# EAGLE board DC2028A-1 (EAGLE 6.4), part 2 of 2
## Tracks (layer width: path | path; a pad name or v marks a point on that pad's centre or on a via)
+3V3  (via drill 0.25)
  Top 0.203: R35.1 61.63,5.5 61.47,5.71 59.56,5.71 59.56,7.49 59.33,7.47 R24.R1_2 | U8.8 59.52,12.99 59.56,12.95 v58.67,12.95 | 66.42,11.81 U13.18 | R25.1 71.63,7.87 71.63,7.37 71.37,7.11 69.98,7.11 69.72,7.37 69.72,10.67 69.09,11.3 69.09,12.19 | C18.2 45.81,19.52 v45.85,19.56 | v45.85,19.56 45.85,20.2 U6.16 | U6.17 45.9,19.5 v45.85,19.56 | v45.85,19.56 45.85,19.5
  Top 0.305: U8.8 59.82,12.95 59.82,11.94 59.8,11.92 59.5,11.92 C20.1 R24.R4_2
  Top 0.406: R24.R1_2 R24.R2_2 R24.R3_2 R24.R4_2 | 66.42,11.81 66.8,12.19 69.09,12.19 69.09,12.83 v69.34,13.08 | R23.2 R22.2 R18.2 57.37,19.47 v57.15,19.68
  Route15 0.406: v69.34,13.08 69.34,12.7 68.96,12.32 67.82,12.32 67.44,11.94 60.81,11.94 U8.8 58.72,12.99 v58.67,12.95 | v24.38,19.94 24.38,17.78 24.51,17.65 45.47,17.65 45.85,18.03 v45.85,19.56
  Bottom 0.203: R60.1 R58.1 68.71,16.6 68.71,14.86 | 68.71,14.86 69.34,14.22 v69.34,13.08 | R67.1 23.07,25.78 | R57.1 67.4,14.31 67.44,14.35 67.44,14.86 68.71,14.86
  Bottom 0.406: v58.67,12.95 58.67,13.59 57.02,15.24 56.32,15.24 R59.R1_2 R59.R2_2 R59.R3_2 R59.R4_2 56.64,17.91 57.15,18.41 v57.15,19.68 57.15,20.32 57.02,20.45 55.88,20.45 55.37,19.94 45.85,19.94 v45.85,19.56 | U16.5 19.81,23.62 19.56,23.88 19.56,25.78 C46.1 23.07,25.78 | R62.2 23.33,20.49 | R62.2 23.37,20.57 | 24.38,20.45 24.51,20.45 24.51,25.27 24.26,25.53 23.41,25.53 R67.1 | v24.38,19.94 24.38,20.45 | R62.2 23.2,20.45 23.2,20.41 23.24,20.45 24.38,20.45
+12V
  Route15 1.016: JP2.14 JP2.13
  pour Top (no thermals): 63.63,30.3 63.63,32.77 72.64,32.77 73.66,33.78 76.07,33.78 77.34,32.64 77.34,30.23 75.82,28.7 68.58,28.7 68.58,29.59 67.82,30.35 65.53,30.35
  pour Bottom (no thermals): 70.61,26.42 70.61,36.45 71.25,37.08 71.25,41.78 71.63,42.16 73.41,42.16 73.79,41.78 73.79,34.29 74.17,33.91 76.07,33.91 77.22,32.89 77.22,30.1 75.56,28.45 75.56,21.08 73.03,18.54 73.03,3.81 72.52,3.3 70.36,3.3 70.36,23.88 72.64,23.88 72.64,26.42
A0_MUX  (via drill 0.25)
  Top 0.203: U13.3 63.37,8.76 62.94,8.38 62.79,8.38 v62.79,8.46 62.79,8.41 62.76,8.38 62.34,8.38 | 62.34,8.38 R24.R2_1 62.08,8.36 62.1,8.38 62.34,8.38
  Bottom 0.203: v62.79,8.46 62.79,8.41 62.76,8.38 61.98,8.38 61.47,7.87 JP3.6
A1_MUX  (via drill 0.25)
  Top 0.203: U13.2 64.16,9.27 63.42,9.27 63.28,9.16 R24.R3_1 61.61,9.16 61.59,9.14 62.79,9.14 | 62.79,9.14 62.9,9.16 | 62.79,9.14 v62.79,9.45 62.79,9.27
  Bottom 0.203: v62.79,9.45 61.9,9.45 61.59,9.14 JP3.7
A2_MUX  (via drill 0.25)
  Top 0.203: 62.79,10.16 63.88,10.16 63.88,9.78 64.14,9.78 U13.1 | R24.R4_1 61.94,10.12 61.98,10.16 62.79,10.16 | 62.79,10.16 v62.79,10.54
  Bottom 0.203: v62.79,10.54 60.71,10.54 JP3.8
ALERTB  (via drill 0.25)
  Top 0.203: v58.42,16.51 58.42,15.11 58.04,14.73 55.63,14.73 | 55.63,14.73 54.48,14.73 53.85,15.37 53.85,16.13 52.7,17.27 v52.32,17.27 52.54,17.31 U6.29 | 55.63,15.62 55.65,15.6 | 55.63,14.73 55.63,15.62 | 55.63,15.62 R23.1
  Route15 0.203: v21.21,18.92 21.21,16.76 48.64,16.76 48.9,17.02 51.05,17.02 51.31,17.27 v52.32,17.27
  Bottom 0.203: JP1.3 62.04,38.42 61.72,38.1 60.58,38.1 59.05,36.58 59.05,33.53 58.93,33.4 58.93,20.95 59.82,20.07 59.82,16.51 | 59.82,16.51 59.82,14.61 60.2,14.22 60.2,12.19 60.45,11.94 62.48,11.94 63.63,10.79 63.63,8.26 61.98,6.6 61.98,3.78 JP2.3 | v58.42,16.51 59.82,16.51 | TP10.TP 15.49,26.92 16.38,26.04 16.38,23.37 16.76,22.99 18.31,22.99 U16.1 18.54,22.99 18.58,22.95 18.58,20.41 20.07,18.92 v21.21,18.92 20.95,18.92
CH7_SHORT  (via drill 0.25)
  Top 0.406: v13.59,24 13.59,18.72 SW2.SW1
  Route15 0.203: v13.59,24 13.59,23.62 8,23.62 6.6,22.23 6.6,16.89 9.27,14.22 12.06,14.22 13.46,15.62 48.51,15.62 49.28,14.86 v51.31,14.86
  Bottom 0.203: Q5.1 53.07,13.1 52.45,13.72 51.56,13.72 51.31,13.97 v51.31,14.86
  Bottom 0.406: R68.2 13.59,25.27 v13.59,24 13.59,19.94 R61.2
CTRL  (via drill 0.25)
  Top 0.203: C26.1 70.74,10.03 71.12,10.41 72.52,10.41 72.77,10.67 S1.5 | U6.31 U6.30 | U6.31 53.34,19.43 | 54.74,18.54 54.74,19.56 54.86,19.68 55.37,19.68 56.01,20.32 56.26,20.32 56.77,20.83 v57.91,20.83 | U6.31 53.41,19.5 53.34,19.43 53.34,18.54 54.74,18.54 | R22.1 54.74,17.14 54.74,18.54
  Top 0.406: S1.2 S1.5
  Route15 0.203: S1.5 | v58.8,18.8 59.18,18.41 59.18,17.27 60.71,15.75 65.15,15.75 65.79,16.38 72.39,16.38 72.77,16 S1.2
  Bottom 0.203: R88.2 59.48,42.08 58.93,41.53 58.93,41.15 | 58.93,41.15 60.02,41.15 JP1.2 58.94,41.13 58.93,41.15 | 58.93,41.15 58.93,37.72 58.29,37.08 58.29,34.04 58.17,33.78 58.17,20.95 58.04,20.83 | 58.04,18.8 58.04,18.54 57.4,17.91 57.4,15.75 59.44,13.72 59.44,12.45 59.18,12.19 59.18,5.21 58.8,4.83 58.8,2.03 59.05,1.78 59.98,1.78 JP2.2 | 58.04,18.8 58.04,20.83 | 58.04,20.83 v57.91,20.83 | 58.04,18.8 v58.8,18.8
CTRL_P
  Bottom 0.203: R88.1 61.17,43.22 61.21,43.18 66.04,43.18 67.03,42.19 67.03,38.38 68.33,37.08 TP8.TP
DACP_CH0  (via drill 0.25)
  Top 0.203: U6.39 55.49,23.25 v55.75,22.99
  Route15 0.203: v55.75,22.99 55.24,22.99 54.99,23.24 54.99,23.5 54.99,23.88 53.59,25.27 48.39,25.27 47.5,26.16 42.67,26.16 41.4,27.43 33.53,27.43 32.77,28.19 32.77,30.61 31.88,31.5 21.97,31.5 21.72,31.75 VSNSN23.1
  Bottom 0.203: R78.2 21.97,33.91 21.72,33.91
  Bottom 0.406: VSNSN23.1 21.72,33.91
DACP_CH1  (via drill 0.25)
  Top 0.203: U6.40 55.63,23.75 v55.75,23.88
  Route15 0.203: v55.75,23.88 53.98,25.65 48.64,25.65 47.75,26.54 42.93,26.54 41.66,27.81 33.78,27.81 33.27,28.32 VSNSN21.1
  Bottom 0.203: R76.2 33.53,33.91 33.27,33.91
  Bottom 0.406: VSNSN21.1 33.27,33.91
DACP_CH2  (via drill 0.25)
  Top 0.203: U6.44 55.27,25.75 55.37,25.65 56.64,25.65 56.77,25.53 v56.77,25.02
  Route15 0.203: v56.77,25.02 56.77,25.53 56.64,25.65 55.5,25.65 54.61,26.54 49.02,26.54 47.37,28.19 47.37,29.72 VSNSN19.1
  Bottom 0.203: R74.2 45.09,33.91 44.83,33.91
  Bottom 0.406: VSNSN19.1 44.83,33.91
DACP_CH3  (via drill 0.25)
  Top 0.203: U6.50 53.54,29.16 53.72,29.34 55.24,29.34 55.37,29.34 55.63,29.08 55.63,28.7 v55.75,28.7
  Bottom 0.203: R72.2 56.64,33.91 56.39,33.91 | v55.75,28.7 55.63,28.7 55.63,31.88 55.88,32.26 VSNSN17.1
  Bottom 0.406: VSNSN17.1 56.39,33.91
DACP_CH4  (via drill 0.25)
  Top 0.203: U6.55 51.04,29.07 51.31,29.34 52.2,29.34 53.09,30.23 56.13,30.23 57.02,29.34 57.02,28.07 56.64,27.69 v56.64,27.56
  Route15 0.203: v56.64,27.56 56.64,27.43 57.4,26.67 57.4,22.61 55.88,21.08 47.62,21.08 45.72,22.99 43.94,22.99 43.18,22.23 43.18,19.3 43.05,19.18 40.77,19.18 39.5,20.45 26.8,20.45 26.67,20.57 21.08,20.57 20.45,19.94 20.45,17.27 14.22,17.27 v14.22,17.4
  Bottom 0.203: R56.2 13.21,12.45 13.46,12.45 | VSNSN16.1 13.72,17.14 13.97,17.4 v14.22,17.4
  Bottom 0.406: 13.46,12.45 13.72,12.45 VSNSN16.1
DACP_CH5  (via drill 0.25)
  Top 0.203: U6.56 50.54,29.21 51.05,29.72 51.94,29.72 52.83,30.61 56.39,30.61 57.53,29.46 v57.53,27.56
  Route15 0.203: v57.53,27.56 57.53,27.18 57.78,26.92 57.78,22.35 56.13,20.7 47.37,20.7 45.47,22.61 44.2,22.61 43.69,22.1 43.69,19.05 43.31,18.67 40.64,18.67 39.37,19.94 v26.16,19.94
  Bottom 0.203: R54.2 24.77,12.45 25.02,12.45 | v26.16,19.94 26.16,15.24 VSNSN14.1
  Bottom 0.406: 25.02,12.45 VSNSN14.1
DACP_CH6  (via drill 0.25)
  Top 0.203: U6.59 49.04,29.32 48.64,29.72 48.26,29.72 47.75,30.23 45.09,30.23 44.45,29.59 v44.45,29.34 | VSNSN12.1 36.58,18.16 36.58,18.41 36.83,18.67 v37.72,18.67
  Bottom 0.203: R52.2 36.32,12.45 36.58,12.45 | v44.45,29.34 43.43,29.34 42.16,28.07 42.16,25.78 41.91,25.53 39.5,25.53 38.35,24.38 38.35,19.18 37.85,18.67 v37.72,18.67
  Bottom 0.406: 36.58,12.45 VSNSN12.1
DACP_CH7  (via drill 0.25)
  Top 0.203: U6.60 48.54,29.18 48.39,29.34 48.01,29.34 47.5,29.84 45.47,29.84 v45.47,29.59
  Bottom 0.203: R50.2 47.88,12.45 48.13,12.45 | VSNSN10.1 48.13,14.73 47.88,14.99 44.07,14.99 43.81,15.24 43.81,27.56 44.07,27.81 44.7,27.81 45.47,28.57 v45.47,29.59
  Bottom 0.406: 48.13,12.45 VSNSN10.1
EESCL
  Top 0.203: 77.47,6.1 77.22,6.35 R30.1 78.03,6.35 | U14.1 77.81,1.59 78.03,1.78 78.03,6.35 | 78.03,6.35 78.03,6.66 78.61,7.24 78.61,8 78.87,8.26 83.66,8.26 84.17,8.76 84.17,10.29 83.72,10.73 82.01,10.73 J2.11 81.09,9.65
EESDA
  Top 0.203: 77.21,3.43 U14.3 77.21,4.83 R36.1 76.33,4.83 76.33,7.06 76.45,7.19 77.95,7.19 78.11,7.34 78.11,8.26 78.49,8.64 82.9,8.64 83.19,8.89 83.19,9.65 J2.12
EEVCC  (via drill 0.25)
  Top 0.203: 78.81,20.77 78.2,20.77 C15.1
  Top 0.254: U7.8 U7.7
  Top 0.406: R36.2 R30.2 75.44,6.35 | U14.4 74.36,3.49 74.68,3.56 | 74.68,4.79 R36.2 | 74.68,3.56 74.55,3.56 | 74.68,4.79 74.68,4.83 | 74.68,3.56 74.68,4.79 | R36.2 74.68,4.83 | 74.68,4.83 v74.3,4.83 | 75.44,6.35 75.35,6.35 | 75.44,6.35 75.44,7.87 C25.1
  Top 0.813: 83.95,37.85 84.07,37.59 84.07,22.61 83.95,22.48
  Top 1.016: 83.95,37.85 82.9,38.86 79.63,38.86 78.87,39.62 74.8,39.62 73.53,40.89 73.53,42.55 73.15,42.93 66.55,42.93 66.02,42.4 66.02,41.15 JP1.8 | 79.63,22.48 83.95,22.48 | 79.63,22.48 v79.63,21.84 79.63,21.59 78.81,20.77 U7.8 | 79.63,22.48 v79.63,22.99
  Route15 0.406: v68.07,19.56 69.6,19.56 71.88,21.84 v79.63,21.84
  Bottom 0.406: D1.2 68.98,19.8 68.58,19.56 v68.07,19.56
  Bottom 0.813: J2.1 81.01,19.7 80.99,19.68 79.6,19.68 arc60 79.63,19.81 v79.63,21.84 v79.63,22.99
  pour Bottom (no thermals): 65.28,2.92 72.77,2.92 73.53,3.68 73.53,18.29 76.07,20.83 81.88,20.83 81.88,18.92 77.72,18.92 75.31,16.51 75.31,0.76 65.28,0.76
  pour Top (no thermals): 75.69,21.46 78.61,21.46 78.99,21.84 78.99,23.5 80.39,23.5 80.39,21.72 78.87,20.19 75.69,20.19
FAULTB  (via drill 0.25)
  Top 0.203: TP9.TP 9.27,31.37 11.68,28.96 11.68,25.15 12.06,24.77 16.89,24.77 v17.38,24.27 | U6.24 U6.23 | U6.24 50.04,19.31 50.04,19.3 v50.04,17.91 50.04,16 50.29,15.75 v50.29,15.49 | U6.24 U6.25 U6.26
  Route15 0.203: v50.29,15.49 57.15,15.49 57.78,16.13 57.78,16.89 58.17,17.27 58.17,19.18 58.67,19.68 v58.8,19.68 | v21.21,19.81 21.84,19.18 21.84,17.27 21.97,17.14 48.39,17.14 48.64,17.4 49.91,17.4 50.04,17.53 v50.04,17.91
  Bottom 0.203: JP2.1 59.78,3.72 59.69,3.81 59.69,6.35 59.56,6.48 59.56,11.94 59.82,12.19 59.82,13.97 57.78,16 57.78,17.65 58.17,18.03 58.93,18.03 59.44,18.54 59.44,19.3 59.05,19.68 v58.8,19.68 58.55,19.68 58.55,33.66 58.67,33.78 58.67,36.83 60.07,38.23 60.07,39.13 JP1.1 | v17.38,24.27 U16.3 18.91,24.27 19.05,24.13 19.05,20.57 19.81,19.81 v21.21,19.81 20.95,19.81 | R59.R2_1 53.58,16.24 52.83,15.49 v50.29,15.49
FB_LTC3604
  Top 0.203: 67.22,23.75 R14.2 67.35,24.42 67.56,24.64 68.2,24.64 68.45,24.89 68.45,27.05 68.2,27.3 68.2,28.96 67.8,29.44 U5.11
  Top 0.305: R15.1 C14.1 67.22,23.75 | R14.2 C11.2
GND  (via drill 0.25)
  Top 0.203: v12.57,32.64 v13.59,32.64 | v13.59,32.64 C5.2 | v13.59,32.64 v14.61,32.64 | v13.59,32.64 13.59,34.16 | R5.1 20.74,39.97 20.83,40.26 | v24.13,32.64 v25.15,32.64 | v25.15,32.64 C6.2 | v25.15,32.64 v26.16,32.64 | v25.15,32.64 25.15,34.16 | R6.1 32.3,39.97 32.38,40.26 | v35.69,32.64 v36.7,32.64 | v36.7,32.64 C7.2 | v36.7,32.64 v37.72,32.64 | v36.7,32.64 36.7,34.16 | R7.1 43.85,39.97 43.94,40.26 | v47.24,32.64 v48.26,32.64 | v48.26,32.64 C8.2 | v48.26,32.64 v49.28,32.64 | v48.26,32.64 48.26,34.16 | R8.1 55.41,39.97 55.5,40.26 | v21.59,13.72 v22.61,13.72 | C21.2 v21.59,13.72 | v21.59,13.72 v20.57,13.72 | v21.59,13.72 21.59,12.2 | R31.1 14.44,6.39 14.35,6.1 | v33.15,13.72 v34.16,13.72 | C22.2 v33.15,13.72 | v33.15,13.72 v32.13,13.72 | v33.15,13.72 33.15,12.2 | R32.1 26,6.39 25.91,6.1 | v44.7,13.72 v45.72,13.72 | C23.2 v44.7,13.72 | v44.7,13.72 v43.69,13.72 | v44.7,13.72 44.7,12.2 | R33.1 37.55,6.39 37.47,6.1 | R34.1 49.11,6.39 49.02,6.1 | v56.26,13.72 v57.28,13.72 | C24.2 v56.26,13.72 | v56.26,13.72 v55.24,13.72 | v56.26,13.72 56.26,12.2 | 48.9,31.37 49.02,31.37 49.53,30.86 49.53,28.52 U6.58 | U6.57 50.04,29.47 50.8,30.23 50.8,30.99 50.16,31.75
  Top 0.305: LED3.N 61.1,17.03 61.34,17.27 61.34,19.43 61.59,19.68 v62.1,19.68
  Top 0.406: 20.83,40.26 20.7,40.13 20.45,40.13 | v19.68,40.13 20.74,40.13 R5.1 | 32.38,40.26 32.26,40.13 32,40.13 | v31.24,40.13 32.3,40.13 R6.1 | 43.94,40.26 43.81,40.13 43.56,40.13 | v42.8,40.13 43.85,40.13 R7.1 | 55.5,40.26 55.37,40.13 55.12,40.13 | v54.36,40.13 55.41,40.13 R8.1 | 14.35,6.1 14.48,6.22 14.73,6.22 | v15.49,6.22 14.44,6.22 R31.1 | 25.91,6.1 26.04,6.22 26.29,6.22 | v27.05,6.22 26,6.22 R32.1 | 37.47,6.1 37.59,6.22 37.85,6.22 | v38.61,6.22 37.55,6.22 R33.1 | 49.02,6.1 49.15,6.22 49.4,6.22 | v50.16,6.22 49.11,6.22 R34.1
  Bottom 0.203: 62.36,19.81 62.61,20.32 | Q9.2 12.19,43.32 | 12.19,43.32 12.19,43.31 | 12.19,43.32 v12.19,44.07 | Q8.2 23.75,43.32 | 23.75,43.32 23.75,43.31 | 23.75,43.32 v23.75,44.07 | Q7.2 35.31,43.32 | 35.31,43.32 35.31,43.31 | 35.31,43.32 v35.31,44.07 | Q6.2 46.86,43.32 | 46.86,43.32 46.86,43.31 | 46.86,43.32 v46.86,44.07 | 22.99,3.03 Q4.2 | 22.99,3.03 22.99,3.05 | v22.99,2.29 22.99,3.03 | 34.54,3.03 Q3.2 | 34.54,3.03 34.54,3.05 | v34.54,2.29 34.54,3.03 | 46.1,3.03 Q2.2 | 46.1,3.03 46.1,3.05 | v46.1,2.29 46.1,3.03 | 57.66,3.03 Q1.2 | 57.66,3.03 57.66,3.05 | v57.66,2.29 57.66,3.03 | 48.9,31.37 49.02,31.37 49.53,30.86 49.53,26.8 50.42,26.8 | 48.48,26.67 47.88,26.67 47.62,26.92 47.62,29.08 48.26,29.72 48.26,31.75 48.51,32 50.04,32 50.16,31.88 50.16,31.75
  Bottom 0.406: 79.72,7.34 79.72,17.78 81.14,17.78 J2.3
  other vias: 66.42,8.76 63.75,14.61 68.2,14.22 65.28,29.21 81.03,7.49 75.56,2.54 73.28,4.57 59.94,25.02 59.94,26.04 71.25,18.29 78.61,18.03 69.34,25.15 70.48,25.15 71.63,25.15 38.99,18.67 47.12,24.51 47.12,23.5 53.59,22.35 43.69,31.5
  pour Top (no thermals): 57.91,14.35 11.81,14.35 11.81,0.76 1.78,0.76 0.89,1.65 0.89,45.59 11.81,45.59 11.81,32 58.93,32 58.93,26.42 60.07,26.42 60.33,26.16 60.33,19.18 80.9,19.18 80.9,22.99 83.57,22.99 83.57,27.56 77.85,27.56 77.85,32.77 76.2,34.29 73.41,34.29 72.39,33.27 63.12,33.27 63.12,32.38 58.93,32.38 58.93,32.13 57.78,32.13 57.78,45.59 84.42,45.59 84.42,0.76 58.04,0.76 57.91,6.35 58.29,6.35 58.29,11.05 57.91,11.05
  pour Route2 (no thermals): 0.89,45.59 0.89,3.05 3.17,0.76 84.42,0.76 84.42,45.59
  pour Bottom (no thermals): 11.94,32 57.66,32 57.78,41.27 58.42,41.27 58.42,44.45 57.66,44.45 57.66,45.59 84.42,45.59 84.42,0.76 75.82,0.76 75.82,16.38 77.85,18.41 82.26,18.41 82.3,21.21 80.39,21.21 80.39,23.37 83.57,23.37 83.57,27.56 79.25,27.56 79.25,21.34 76.07,21.34 76.07,28.19 77.72,29.84 77.72,33.15 76.33,34.42 74.42,34.42 74.3,34.54 74.3,41.91 73.53,42.67 71.5,42.67 70.87,42.04 70.87,37.34 70.23,36.7 70.23,25.91 72.14,25.91 72.14,24.38 69.85,24.38 69.85,3.3 64.9,3.3 64.9,0.76 58.04,0.76 58.04,11.18 57.78,11.18 57.78,13.84 58.04,13.84 58.04,14.35 11.81,14.35 11.81,5.08 11.3,5.08 11.3,1.78 11.81,1.78 11.81,0.76 0.89,0.76 0.89,45.59 11.81,45.59 11.68,35.56 11.94,35.31
  pour Top (no thermals): 64.52,29.84 67.69,29.84 68.2,29.34 68.2,28.19 76.07,28.19 77.85,29.97 77.85,27.56 72.01,27.56 72.01,24.26 76.83,24.26 77.6,23.5 78.49,23.5 78.49,21.97 78.36,21.84 65.28,21.84 65.28,25.02 64.52,25.02
  pour Bottom (no thermals): 23.37,41.27 23.37,36.58 21.21,36.58 20.83,36.2 20.83,35.05 18.92,35.05 18.92,36.58 19.3,36.96 19.3,40.26 20.32,41.27
  pour Top (no thermals): 15.62,32 11.94,32 11.94,35.31 16.89,35.31 17.53,34.67 17.53,33.02 16.89,33.02 16.89,34.42 16.64,34.67 15.88,34.67 15.62,34.42
  pour Bottom (no thermals): 15.62,32 12.06,32 12.06,35.18 15.24,35.18 15.62,34.8
  pour Bottom (no thermals): 34.92,41.27 34.92,36.58 32.77,36.58 32.38,36.2 32.38,35.05 30.48,35.05 30.48,36.58 30.86,36.96 30.86,40.26 31.88,41.27
  pour Top (no thermals): 27.18,32 23.62,32 23.62,35.31 28.45,35.31 29.08,34.67 29.08,33.02 28.45,33.02 28.45,34.42 28.19,34.67 27.43,34.67 27.18,34.42
  pour Bottom (no thermals): 27.18,32 23.62,32 23.62,35.18 26.8,35.18 27.18,34.8
  pour Bottom (no thermals): 46.48,41.27 46.48,36.58 44.32,36.58 43.94,36.2 43.94,35.05 42.04,35.05 42.04,36.58 42.42,36.96 42.42,40.26 43.43,41.27
  pour Top (no thermals): 38.73,32 35.18,32 35.18,35.31 40.01,35.31 40.64,34.67 40.64,33.02 40.01,33.02 40.01,34.42 39.75,34.67 38.99,34.67 38.73,34.42
  pour Bottom (no thermals): 38.73,32 35.18,32 35.18,35.18 38.35,35.18 38.73,34.8
  pour Bottom (no thermals): 58.04,41.27 58.04,36.58 55.88,36.58 55.5,36.2 55.5,35.05 53.59,35.05 53.59,36.58 53.98,36.96 53.98,40.26 54.99,41.27
  pour Top (no thermals): 50.29,32 46.74,32 46.74,35.31 51.56,35.31 52.2,34.67 52.2,33.02 51.56,33.02 51.56,34.42 51.31,34.67 50.55,34.67 50.29,34.42
  pour Bottom (no thermals): 50.29,32 46.74,32 46.74,35.18 49.91,35.18 50.29,34.8
  pour Top (no thermals): 19.56,14.35 23.11,14.35 23.11,11.05 18.29,11.05 17.65,11.68 17.65,13.34 18.29,13.34 18.29,11.94 18.54,11.68 19.3,11.68 19.56,11.94
  pour Bottom (no thermals): 19.56,14.35 23.11,14.35 23.11,11.18 19.94,11.18 19.56,11.56
  pour Bottom (no thermals): 11.81,5.08 11.81,9.78 13.97,9.78 14.35,10.16 14.35,11.3 16.26,11.3 16.26,9.78 15.88,9.4 15.88,6.1 14.86,5.08
  pour Top (no thermals): 31.11,14.35 34.67,14.35 34.67,11.05 29.84,11.05 29.21,11.68 29.21,13.34 29.84,13.34 29.84,11.94 30.1,11.68 30.86,11.68 31.11,11.94
  pour Bottom (no thermals): 31.11,14.35 34.67,14.35 34.67,11.18 31.5,11.18 31.11,11.56
  pour Bottom (no thermals): 23.62,5.08 23.62,6.73 24,7.11 24,9.78 25.53,9.78 25.91,10.16 25.91,11.3 27.81,11.3 27.81,9.78 27.43,9.4 27.43,6.1 26.42,5.08
  pour Top (no thermals): 42.67,14.35 46.23,14.35 46.23,11.05 41.4,11.05 40.77,11.68 40.77,13.34 41.4,13.34 41.4,11.94 41.66,11.68 42.42,11.68 42.67,11.94
  pour Bottom (no thermals): 42.67,14.35 46.23,14.35 46.23,11.18 43.05,11.18 42.67,11.56
  pour Bottom (no thermals): 35.18,5.08 35.18,6.73 35.56,7.11 35.56,9.78 37.08,9.78 37.47,10.16 37.47,11.3 39.37,11.3 39.37,9.78 38.99,9.4 38.99,6.1 37.97,5.08
  pour Top (no thermals): 54.23,14.35 57.78,14.35 57.78,11.05 52.96,11.05 52.32,11.68 52.32,13.34 52.96,13.34 52.96,11.94 53.21,11.68 53.98,11.68 54.23,11.94
  pour Bottom (no thermals): 54.23,14.35 57.78,14.35 57.78,11.18 54.61,11.18 54.23,11.56
  pour Bottom (no thermals): 46.74,5.08 46.74,6.73 47.12,7.11 47.12,9.78 48.64,9.78 49.02,10.16 49.02,11.3 50.93,11.3 50.93,9.78 50.55,9.4 50.55,6.1 49.53,5.08
IBV_AUX  (via drill 0.25)
  Top 0.203: C11.1 64.17,24.42 64.34,24.59 66.24,24.59 66.8,25.15 66.8,26.04 65.91,26.92 65.91,27.34 U5.8 | 61.73,27.51 61.73,25.02 | U7.1 70.96,20.77 C16.1 | v67.18,21.21 67.18,21.03 67.94,20.77
  Top 0.254: U7.1 U7.2
  Top 0.406: C11.1 64.05,23.75 R15.2 62.48,22.23 61.85,22.23 61.85,22.99 C13.1 61.72,22.99 61.73,27.51 L5.2
  Top 1.016: 66.88,20.77 67.94,20.77 U7.1 | 62.48,22.23 62.48,21.72 63.68,20.77 66.88,20.77 | R17.2 66.97,20.73 66.93,20.83 66.88,20.77
  Bottom 0.406: D1.1 67.2,21.1 v67.18,21.21
  pour Top (no thermals): 60.83,19.81 60.83,26.42 60.45,26.8 59.44,26.8 59.44,28.32 61.59,28.32 62.1,27.81 62.1,24.51 64.77,24.51 64.77,21.46 73.15,21.46 73.15,19.94 73.03,19.81
INTVCC_LTC3604  (via drill 0.25)
  Top 0.203: v66.04,25.73 66.04,26.16 65.41,26.8 65.41,27.33 U5.7 | U5.1 62.77,29.94 62.74,29.97 v62.74,30.61 | U5.10 67.58,28.94 67.69,28.83 v67.69,25.4
  Bottom 0.203: C47.1 68.96,27.22 68.92,27.18 67.69,27.18 | 66.04,27.18 v66.04,25.73 | 66.04,27.18 62.87,27.18 62.74,27.3 v62.74,30.61 | 66.04,27.18 67.69,27.18 | 67.69,27.18 v67.69,25.4
ITH_LTC3604  (via drill 0.25)
  Top 0.203: U5.12 67.66,29.94 67.82,30.1 v67.82,30.86
  Bottom 0.203: v67.82,30.86 67.56,30.86 67.56,28.83 66.55,28.83 | 66.51,28.83 R71.2 66.55,28.83 | C48.1 64.26,28.57 66.55,28.57 66.55,28.83
N$1
  Bottom 0.406: D1.3 66.8,20.45 66.04,21.21 C42.1 65.15,21.34 64.52,21.97 64.52,24.26 64.71,24.45 U15.4
N$3  (via drill 0.25)
  Top 0.203: v22.1,24.51 LED1.P
  Bottom 0.203: v22.1,24.51 22.1,24 22.31,23.79 23.33,23.79 23.37,23.75 R67.2
N$4  (via drill 0.25)
  Top 0.203: U13.16 68.2,11.01 v68.2,11.43
  Route15 0.203: v68.2,11.43 60.45,11.43 59.56,12.32 58.42,12.32 57.91,12.83 57.91,14.22 57.4,14.73 54.48,14.73 54.1,14.35 54.1,13.59 53.47,12.95 48.13,12.95 46.23,14.86 16.76,14.86 v16.76,14.48
  Bottom 0.203: R61.1 15.33,15.91 15.88,15.37 16.51,15.37 16.76,15.11 v16.76,14.48
N$6
  Top 0.406: P1.P 12.19,43.05 12.19,40.77 12.95,40.77 R9.1
N$7  (via drill 0.25)
  Top 0.203: v15.49,43.69 15.11,43.31 14.59,43.31 P1.N
  Bottom 0.203: v15.49,43.69 14.22,43.69 14.22,42.67 Q9.3
N$8
  Top 0.406: P2.P 23.75,43.05 23.75,40.77 24.51,40.77 R10.1
N$9  (via drill 0.25)
  Top 0.203: v27.05,43.69 26.67,43.31 26.15,43.31 P2.N
  Bottom 0.203: v27.05,43.69 25.78,43.69 25.78,42.67 Q8.3
N$10
  Top 0.406: P3.P 35.31,43.05 35.31,40.77 36.07,40.77 R11.1
N$11  (via drill 0.25)
  Top 0.203: v38.61,43.69 38.23,43.31 37.71,43.31 P3.N
  Bottom 0.203: v38.61,43.69 37.34,43.69 37.34,42.67 Q7.3
N$12
  Top 0.406: P4.P 46.86,43.05 46.86,40.77 47.62,40.77 R12.1
N$13  (via drill 0.25)
  Top 0.203: v50.16,43.69 49.78,43.31 49.26,43.31 P4.N
  Bottom 0.203: v50.16,43.69 48.9,43.69 48.9,42.67 Q6.3
N$16
  Bottom 0.203: R57.2 67.06,9.65 67.44,9.27 67.44,6.73 67.56,6.6 JP3.4
N$29
  Top 0.406: P5.P 22.99,3.3 22.99,5.59 22.23,5.59 R26.1
N$30  (via drill 0.25)
  Top 0.203: v19.68,2.67 20.07,3.05 20.59,3.05 P5.N
  Bottom 0.203: v19.68,2.67 20.95,2.67 20.95,3.68 Q4.3
N$31
  Top 0.406: P6.P 34.54,3.3 34.54,5.59 33.78,5.59 R27.1
N$32  (via drill 0.25)
  Top 0.203: v31.24,2.67 31.62,3.05 32.14,3.05 P6.N
  Bottom 0.203: v31.24,2.67 32.51,2.67 32.51,3.68 Q3.3
N$33
  Top 0.406: P7.P 46.1,3.3 46.1,5.59 45.34,5.59 R28.1
N$34  (via drill 0.25)
  Top 0.203: v42.8,2.67 43.18,3.05 43.7,3.05 P7.N
  Bottom 0.203: v42.8,2.67 44.07,2.67 44.07,3.68 Q2.3
N$35
  Top 0.406: P8.P 57.66,3.3 57.66,5.59 56.9,5.59 R29.1
N$36  (via drill 0.25)
  Top 0.203: v54.36,2.67 54.74,3.05 55.26,3.05 P8.N
  Bottom 0.203: v54.36,2.67 55.63,2.67 55.63,3.68 Q1.3
N$53
  Top 0.203: U6.35 54.86,21.21 55.75,21.21 56.39,21.84 56.39,23.5 57.15,23.5 C12.1
N$54
  Top 0.203: U6.34 55.93,20.75 56.9,21.72 56.9,22.23 C12.2
N$56
  Top 0.203: U6.18 46.99,19.5 46.99,17.82 C19.2
N$57  (via drill 0.25)
  Top 0.203: v22.1,22.23 LED2.P
  Bottom 0.203: v22.1,22.23 23.37,22.23 R62.1
N$58  (via drill 0.25)
  Top 0.203: LED1.N 24.38,24.51 24.38,24 24.13,23.75 22.35,23.75 22.1,23.5 v22.1,23.11
  Bottom 0.203: v22.1,23.11 21.72,23.11 21.34,23.5 21.34,24 21.08,24.26 20.57,24.26 20.57,24.31 U16.4
N$60  (via drill 0.25)
  Top 0.203: LED2.N 24.38,22.23 24.38,21.59 24.13,21.34 v22.1,21.34
  Bottom 0.203: v22.1,21.34 21.84,21.34 21.46,21.72 21.46,22.61 21.08,22.99 20.55,22.99 U16.6
N$61
  Bottom 0.203: 66.55,31.46 C49.1
  Bottom 0.406: R71.1 66.55,31.46
N$63
  Top 0.305: R16.1 59.94,20.7 LED3.P
N$64  (via drill 0.25)
  Top 0.203: R21.2 75.69,18.33 75.69,18.92 75.18,19.43 v74.8,19.43 74.67,19.43 U7.5
  Route15 0.203: v74.8,19.43 70.23,19.43 69.72,18.92 67.69,18.92 67.44,19.18 67.44,19.94 67.82,20.32 68.96,20.32 70.1,21.46 v70.1,22.35
  Bottom 0.203: v70.1,22.35 R63.1
N$66
  Top 0.203: U13.4 63.58,8.29 62.99,7.7 62.99,7.24 62.48,6.73 62.48,5.08 62.74,4.83 66.17,4.83 66.4,4.65 66.88,4.65 68.2,5.97 69.34,5.97 69.98,5.33 72.3,5.33 C27.1 72.3,6.39 72.26,6.48 | 73.75,7.75 R25.2
  Top 0.254: 72.26,6.48 72.77,6.48 72.77,6.99 73.41,7.62 73.41,7.75 73.75,7.75
N$68
  Top 0.203: U7.4 74.17,19.56 74.17,18.29 74.17,18.33 R20.2
N$69
  Top 0.203: U7.6 75.17,20.08 75.56,19.68 76.2,19.68 76.58,19.3 76.58,17.4 76.45,17.27 73.41,17.27 73.28,17.4 73.28,19.18 | U7.3 73.67,19.44 73.41,19.18 73.28,19.18 | 73.28,19.18 69.09,19.18 68.83,18.92 68.83,18.41 68.45,18.41 68.45,18.33 R19.2 68.49,18.29 | R17.1 66.93,18.29
  Top 0.406: 66.93,18.29 R19.2
N$70
  Top 0.203: 64.66,25.63 64.66,25.59 C10.2 64.64,25.49 64.64,25.65 | 64.64,25.65 64.77,25.65 | 64.64,25.65 64.64,26.7 64.94,27 U5.6
N$74  (via drill 0.25)
  Top 0.203: R35.2 63.37,5.84 63.37,5.46 66.55,5.46 | 66.55,5.46 v66.55,5.33 | 66.55,5.46 66.8,5.46 66.93,5.59 U13.9 | U8.1 65.95,12.99 66.04,13.08 v66.04,13.34
  Bottom 0.203: v66.04,13.34 66.04,10.03 67.06,9.02 67.06,5.71 66.93,5.46 66.55,5.46 v66.55,5.33
RESETB  (via drill 0.25)
  Top 0.203: v49.4,15.75 49.15,15.75 49.15,17.53 49.15,18.54 49.15,18.8 49.02,18.92 49.02,19.48 U6.22 | SW1.SW1 13.59,27.56 v13.59,28.83
  Route15 0.203: v62.1,16.38 60.71,16.38 59.69,17.4 59.69,18.67 59.44,18.92 59.44,20.19 59.18,20.45 58.42,20.45 58.17,20.19 58.17,19.81 57.78,19.43 57.78,17.53 57.4,17.14 57.4,16.38 56.9,15.88 50.8,15.88 50.55,16.13 49.4,16.13 49.4,16 | v13.59,28.83 13.59,25.15 14.48,24.26 14.48,23.75 13.84,23.11 8.13,23.11 7.11,22.1 7.11,17.14 9.65,14.61 11.81,14.61 13.21,16 49.4,16 | 49.4,16 v49.4,15.75
  Bottom 0.203: 62.1,15.88 62.23,15.88 62.36,15.75 65.15,15.75 66.04,16.64 66.04,17.27 66.29,17.53 67.56,17.53 67.82,17.27 67.82,15.88 67.06,15.11 66.29,15.11 65.28,14.1 65.28,12.7 65.66,12.32 65.66,5.08 66.02,4.71 66.04,4.69 JP2.7 | 62.1,15.88 61.59,15.88 61.34,16.13 61.34,19.81 61.59,20.07 61.59,31.88 62.87,31.88 65.15,34.16 65.15,37.34 66.04,38.23 JP1.7 | v62.1,16.38 62.1,15.88 | R59.R3_1 53.61,17.04 52.58,16 50.8,16 50.67,16.13 49.78,16.13 v49.4,15.75
  Bottom 0.406: v13.59,28.83 C44.1
RUN_CH0
  Top 0.203: U1.1 16.38,33.78 16.44,33.73 16.44,32.33 VSNSN1.1 16.51,31.75 16.76,31.5 41.91,31.5 42.42,30.99 42.42,27.3 43.43,26.29 45.76,26.29 U6.4
  Bottom 0.203: R83.1 12.48,38.77 11.81,38.1 11.81,35.94 12.19,35.56 15.62,35.56 16.51,34.67 VSNSN1.1
  Bottom 0.406: Q9.1 12.23,42.02 12.19,41.91 12.19,40.39 R83.1
RUN_CH1  (via drill 0.25)
  Top 0.203: U2.1 27.94,33.78 28,33.73 28,32.33 VSNSN2.1 | v28.07,30.86 28.07,31.11 41.53,31.11 41.91,30.73 41.91,27.18 43.31,25.78 45.76,25.78 U6.5
  Bottom 0.203: R82.1 24.04,38.77 23.37,38.1 23.37,35.94 23.75,35.56 27.18,35.56 28.07,34.67 VSNSN2.1 v28.07,30.86
  Bottom 0.406: Q8.1 23.79,42.02 23.75,41.91 23.75,40.39 R82.1
RUN_CH2  (via drill 0.25)
  Top 0.203: U3.1 39.5,33.78 39.55,33.73 39.55,32.33 VSNSN3.1 | v39.62,30.48 39.62,30.73 41.15,30.73 41.4,30.48 41.4,27.05 43.18,25.27 45.77,25.27 U6.6
  Bottom 0.203: R81.1 35.6,38.77 34.92,38.1 34.92,35.94 35.31,35.56 38.73,35.56 39.62,34.67 VSNSN3.1 v39.62,30.48
  Bottom 0.406: Q7.1 35.34,42.02 35.31,41.91 35.31,40.39 R81.1
RUN_CH3  (via drill 0.25)
  Top 0.203: U4.1 51.05,33.78 51.11,33.73 51.11,32.33 VSNSN4.1 51.56,32.26 v51.56,30.35 | v41.02,26.16 41.02,26.04 41.66,26.04 42.93,24.77 45.78,24.77 U6.7
  Route15 0.203: v51.56,30.35 51.05,29.84 48.51,29.84 47.5,30.86 v47.5,31.24
  Bottom 0.203: R80.1 47.16,38.77 46.48,38.1 46.48,35.94 46.86,35.56 50.29,35.56 51.18,34.67 VSNSN4.1 | v47.5,31.24 44.7,31.24 41.53,28.07 41.53,26.16 v41.02,26.16
  Bottom 0.406: Q6.1 46.9,42.02 46.86,41.91 46.86,40.39 R80.1
RUN_CH4
  Top 0.203: U9.1 18.8,12.57 18.74,12.63 18.74,14.03 VSNSN5.1 19.56,14.99 34.8,14.99 34.92,15.11 34.92,19.18 36.32,20.57 38.1,20.57 38.35,20.83 38.35,24.77 39.12,25.53 41.53,25.53 42.8,24.25 U6.8
  Bottom 0.203: R48.1 22.69,7.58 23.37,8.26 23.37,10.41 22.99,10.79 19.56,10.79 18.67,11.68 VSNSN5.1
  Bottom 0.406: Q4.1 22.95,4.33 22.99,4.45 22.99,5.97 R48.1
RUN_CH5
  Top 0.203: U10.1 30.42,14.03 30.35,14.1 VSNSN6.1 30.73,14.61 35.18,14.61 35.43,14.86 35.43,19.05 36.58,20.19 39.88,20.19 40.51,20.83 41.91,20.83 43.05,21.97 43.05,23.37 43.44,23.75 U6.9
  Bottom 0.203: R47.1 34.25,7.58 34.92,8.26 34.92,10.41 34.54,10.79 31.11,10.79 30.23,11.68 VSNSN6.1
  Bottom 0.406: Q3.1 34.51,4.33 34.54,4.45 34.54,5.97 R47.1
RUN_CH6
  Top 0.203: U11.1 41.98,14.03 41.91,14.1 VSNSN7.1 41.02,14.1 41.02,18.54 40.51,19.05 40.51,20.19 40.77,20.45 42.16,20.45 43.43,21.72 43.43,22.99 43.7,23.25 U6.10
  Bottom 0.203: R46.1 45.81,7.58 46.48,8.26 46.48,10.41 46.1,10.79 42.67,10.79 42.16,11.3 42.16,13.72 VSNSN7.1
  Bottom 0.406: Q2.1 46.06,4.33 46.1,4.45 46.1,5.97 R46.1
RUN_CH7  (via drill 0.25)
  Top 0.203: U12.1 53.54,14.03 53.47,14.1 VSNSN8.1 53.34,14.61 52.96,14.99 52.96,15.37 52.45,15.88 51.44,15.88 51.05,16.26 51.05,17.78 v51.31,18.03 | U6.11 45.1,22.75 44.83,22.48 v44.83,21.59
  Route15 0.203: v51.31,18.03 50.8,18.54 49.53,18.54 48.9,19.18 47.24,19.18 v44.83,21.59
  Bottom 0.203: R45.1 57.37,7.58 58.04,8.26 58.04,10.41 57.66,10.79 54.61,10.79 53.72,11.68 53.72,13.72 VSNSN8.1
  Bottom 0.406: Q1.1 57.62,4.33 57.66,4.45 57.66,5.97 R45.1
SCL  (via drill 0.25)
  Top 0.203: U8.2 64.85,13.59 64.01,13.59 63.25,12.83 62.61,12.83 62.1,13.34 62.1,13.84 61.72,14.22 61.21,14.22 60.83,14.61 60.83,15.11 60.45,15.49 59.05,15.49 58.8,15.24 58.8,14.86 58.29,14.35 54.23,14.35 53.34,15.24 53.34,16 52.7,16.64 v51.69,16.64 51.69,17.53 52.04,17.88 U6.28
  Route15 0.203: v51.69,16.64 51.56,16.51 49.02,16.51 48.9,16.38 13.21,16.38 12.95,16.64 12.95,17.02 12.95,18.92 12.32,19.56 TP13.TP
  Bottom 0.203: R59.R4_1 54.25,17.93 54.23,17.91 | 54.23,17.91 54.23,18.03 | 54.23,17.91 54.23,17.78 53.72,17.78 52.58,16.64 v51.69,16.64
SCL_IN  (via drill 0.25)
  Top 0.203: U8.3 64.6,14.22 67.06,14.22 | J2.4 83.01,17.64 82.11,16.74 80.33,16.74 79.72,16.13 67.06,16.13 67.06,15.62 | 67.06,14.22 67.06,13.21 65.91,12.06 65.91,11.02 U13.19 | v65.91,15.62 67.06,15.62 | 67.06,15.62 67.06,14.22
  Bottom 0.203: 64.77,15.24 62.23,15.24 61.98,15.49 61.21,15.49 60.96,15.75 60.96,20.07 61.21,20.32 61.21,32.26 62.61,32.26 64.64,34.29 64.64,37.59 65.05,37.95 65.05,40.12 JP1.6 | 64.77,15.24 64.77,12.45 65.28,11.94 65.28,5.08 65.05,4.85 65.05,2.18 64.64,1.78 64.08,1.78 64.08,1.72 JP2.6 | 64.77,15.24 65.53,15.24 v65.91,15.62 66.67,16.38 66.8,16.38 66.97,16.42 R58.2
SDA  (via drill 0.25)
  Top 0.203: 59.94,13.59 59.55,13.59 | U8.7 59.89,13.64 59.94,13.59 | 59.94,13.59 60.45,13.59 61.09,12.95 v61.09,12.7 | v52.32,14.86 52.32,15.24 52.07,15.49 51.18,15.49 50.67,16 50.67,18.41 50.93,18.67 51.31,18.67 51.56,18.92 51.56,19.48 U6.27
  Route15 0.203: v61.09,12.7 58.67,15.11 52.32,15.11 v52.32,14.86 52.32,13.46 52.2,13.34 49.28,13.34 49.02,13.59 49.02,14.48 48.26,15.24 13.72,15.24 12.32,13.84 9.78,13.84 9.27,13.34 TP15.TP
  Bottom 0.203: R59.R1_1 53.57,15.34 53.06,14.83 52.43,14.83 v52.32,14.86
SDA_IN  (via drill 0.25)
  Top 0.203: U13.20 65.42,12.05 65.15,12.32 62.48,12.32 61.59,13.21 61.59,13.59 v61.47,13.59 61.21,13.59 60.45,14.35 59.95,14.35 U8.6 | J2.2 83.14,20.46 82.77,20.83 80.23,20.83 79.85,20.45 79.85,17.02 79.47,16.64 66.04,16.64 | v62.87,13.46 62.74,13.72 62.74,14.99 63.25,15.49 64.9,15.49 66.04,16.64 | 66.04,16.64 66.04,17.45 66.09,17.53 66.09,19.68 v65.79,19.68
  Bottom 0.203: JP2.4 63.04,2.72 63.04,6.81 64.14,8 64.14,11.05 62.87,12.32 v62.87,13.46 62.87,13.59 v61.47,13.59 60.96,13.59 60.58,13.97 60.58,14.48 60.2,14.86 60.2,20.32 59.31,21.21 59.31,33.15 59.44,33.27 59.44,36.32 60.83,37.72 62.87,37.72 63.04,37.9 63.04,40.08 62.02,41.1 62.02,41.13 JP1.4
  Bottom 0.254: v65.79,19.68 66.29,19.68 66.67,19.3 66.67,18.41 R60.2
SHARE_CLK  (via drill 0.25)
  Top 0.203: 48.51,19.43 48.57,19.36 | v48.51,18.54 48.51,19.43 | v61.47,14.86 61.47,15.11 60.71,15.88 59.31,15.88 59.05,16.13 59.05,17.53 58.17,18.41 58.17,19.68 57.53,20.32 56.9,20.32 v56.26,19.68 56.26,18.67 R18.1 55.66,19.09 | 48.51,19.43 48.51,19.48 U6.21
  Route15 0.203: v60.45,5.08 60.83,5.08 61.09,4.83 61.21,4.83 63.52,4.83 64.02,4.32 64.02,3.73 JP2.5
  Bottom 0.203: 60.96,14.86 60.96,14.35 61.09,14.22 63.12,14.22 63.5,13.84 63.5,12.32 64.52,11.3 64.52,7.49 64.02,7 64.02,3.72 JP2.5 | 60.96,14.86 v61.47,14.86 | 60.96,14.86 60.58,15.24 60.58,20.32 60.83,20.57 60.83,32.64 62.36,32.64 64.14,34.42 64.14,35.43 | 64.14,35.43 64.14,37.59 64.01,37.72 64.01,39.12 64.02,39.13 JP1.5 | 64.14,35.43 TP7.TP | v48.51,18.54 50.8,18.54 51.44,19.18 56.13,19.18 56.26,19.3 v56.26,19.68 | JP3.5 60.66,5.38 v60.45,5.08
SW1
  pour Top (no thermals): 22.1,33.02 17.91,33.02 17.91,34.67 22.1,34.67
SW2
  pour Top (no thermals): 33.66,33.02 29.46,33.02 29.46,34.67 33.66,34.67
SW3
  pour Top (no thermals): 45.21,33.02 41.02,33.02 41.02,34.67 45.21,34.67
SW4
  pour Top (no thermals): 56.77,33.02 52.58,33.02 52.58,34.67 56.77,34.67
SW11
  pour Top (no thermals): 13.08,13.34 17.27,13.34 17.27,11.68 13.08,11.68
SW12
  pour Top (no thermals): 24.64,13.34 28.83,13.34 28.83,11.68 24.64,11.68
SW13
  pour Top (no thermals): 36.2,13.34 40.39,13.34 40.39,11.68 36.2,11.68
SW14
  pour Top (no thermals): 47.75,13.34 51.94,13.34 51.94,11.68 47.75,11.68
SW_LTC3604
  Top 0.203: 62.93,25.37 C10.1
  pour Top (no thermals): 59.31,28.83 61.72,28.83 62.61,27.94 62.61,24.89 64.14,24.89 64.14,28.96 63.12,28.96 63.12,32 59.31,32
UNUSED1
  Route15 0.203: JP1.9 68.04,38.39 68.33,38.1 74.55,38.1 75.18,38.73 82.93,38.73 83.57,38.1 83.82,37.85 83.82,22.35 82.04,20.57 82.04,19.18 81.58,18.73 80.06,18.73 79.88,18.54 79.88,10.41 77.72,8.26 77.72,6.99 77.34,6.6 68.71,6.6 68.07,5.97 68.07,3.75 JP2.9
UNUSED2  (via drill 0.25)
  Top 0.203: v69.04,5.21 69.04,2.74 JP2.10
  Route15 0.203: JP1.10 68.07,41.13 68.07,41.91 68.58,42.42 73.15,42.42 73.91,41.66 73.91,40.51 75.18,39.24 83.44,39.24 84.33,38.35 84.33,9.4 83.57,8.64 78.87,8.64 78.36,8.13 78.36,6.86 77.6,6.1 69.47,6.1 69.04,5.66 v69.04,5.21
VDD  (via drill 0.25)
  Top 0.203: v14.22,38.61 13.08,38.61 13.08,39.24 13.04,39.12 R9.2 | v25.78,38.61 24.64,38.61 24.64,39.24 24.6,39.12 R10.2 | v37.34,38.61 36.2,38.61 36.2,39.24 36.16,39.12 R11.2 | v48.9,38.61 47.75,38.61 47.75,39.24 47.71,39.12 R12.2 | v55.63,7.75 56.77,7.75 56.77,7.11 56.81,7.24 R29.2 | v44.07,7.75 45.21,7.75 45.21,7.11 45.25,7.24 R28.2 | v32.51,7.75 33.66,7.75 33.66,7.11 33.69,7.24 R27.2 | v20.95,7.75 22.1,7.75 22.1,7.11 22.14,7.24 R26.2 | U6.15 U6.14 | U6.15 44.88,20.75 | U6.15 43.1,20.75 42.55,20.19 42.55,19.9 C17.2 | U7.16 U7.15 73.17,26.44 73.28,26.54 75.56,26.54 75.69,26.42 75.69,25.22 U7.10 U7.9
  Top 0.406: v17.4,18.54 SW2.SW2 | R16.2 62.23,20.7 63.88,19.05 TP14.TP | v41.15,19.81 41.87,19.81 C17.2
  Bottom 0.203: 14.22,40.39 R83.2 | 25.78,40.39 R82.2 | 37.34,40.39 R81.2 | 48.9,40.39 R80.2 | R45.2 55.63,5.97 | 44.07,5.97 R46.2 | R47.2 32.51,5.97 | 20.95,5.97 R48.2
  Bottom 0.406: v14.22,38.61 14.22,40.39 | v25.78,38.61 25.78,40.39 | v37.34,38.61 37.34,40.39 | v48.9,38.61 48.9,40.39 | 55.63,5.97 v55.63,7.75 | v44.07,7.75 44.07,5.97 | 32.51,5.97 v32.51,7.75 | v20.95,7.75 20.95,5.97
  other vias: 82.68,26.04 80.01,24.13 82.68,26.92 82.68,24.13 13.34,41.91 24.89,41.91 36.45,41.91 48.01,41.91 56.52,4.45 44.96,4.45 33.4,4.45 21.84,4.45 82.68,25.02 80.01,25.02 80.01,26.04 80.01,26.92
  pour Route15 (no thermals): 0.89,45.59 0.89,2.29 2.41,0.76 84.42,0.76 84.42,45.59
  pour Bottom (no thermals): 79.63,27.18 83.19,27.18 83.19,23.88 79.63,23.88
  pour Top (no thermals): 18.54,35.69 17.91,35.69 17.91,37.21 17.65,37.47 16.89,37.47 16.64,37.21 16.64,35.69 12.19,35.69 12.19,39.5 13.59,39.5 13.84,39.75 13.84,41.15 13.59,41.4 12.83,41.4 12.83,42.29 14.86,42.29 14.86,39.37 16,38.23 17.78,38.23 18.54,37.47
  pour Top (no thermals): 30.1,35.69 29.46,35.69 29.46,37.21 29.21,37.47 28.45,37.47 28.19,37.21 28.19,35.69 23.62,35.69 23.62,39.5 25.15,39.5 25.4,39.75 25.4,41.15 25.15,41.4 24.38,41.4 24.38,42.29 26.42,42.29 26.42,39.37 27.56,38.23 29.34,38.23 30.1,37.47
  pour Top (no thermals): 41.66,35.69 41.02,35.69 41.02,37.21 40.77,37.47 40.01,37.47 39.75,37.21 39.75,35.69 35.18,35.69 35.18,39.5 36.7,39.5 36.96,39.75 36.96,41.15 36.7,41.4 35.94,41.4 35.94,42.29 37.97,42.29 37.97,39.37 39.12,38.23 40.89,38.23 41.66,37.47
  pour Top (no thermals): 53.21,35.69 52.58,35.69 52.58,37.21 52.32,37.47 51.56,37.47 51.31,37.21 51.31,35.69 46.74,35.69 46.74,39.5 48.26,39.5 48.51,39.75 48.51,41.15 48.26,41.4 47.5,41.4 47.5,42.29 49.53,42.29 49.53,39.37 50.67,38.23 52.45,38.23 53.21,37.47
  pour Top (no thermals): 51.31,10.67 51.94,10.67 51.94,9.14 52.2,8.89 52.96,8.89 53.21,9.14 53.21,10.67 57.78,10.67 57.78,6.86 56.26,6.86 56.01,6.6 56.01,5.21 56.26,4.95 57.02,4.95 57.02,4.06 54.99,4.06 54.99,6.99 53.85,8.13 52.07,8.13 51.31,8.89
  pour Top (no thermals): 39.75,10.67 40.39,10.67 40.39,9.14 40.64,8.89 41.4,8.89 41.66,9.14 41.66,10.67 46.23,10.67 46.23,6.86 44.7,6.86 44.45,6.6 44.45,5.21 44.7,4.95 45.47,4.95 45.47,4.06 43.43,4.06 43.43,6.99 42.29,8.13 40.51,8.13 39.75,8.89
  pour Top (no thermals): 28.19,10.67 28.83,10.67 28.83,9.14 29.08,8.89 29.84,8.89 30.1,9.14 30.1,10.67 34.67,10.67 34.67,6.86 33.15,6.86 32.89,6.6 32.89,5.21 33.15,4.95 33.91,4.95 33.91,4.06 31.88,4.06 31.88,6.99 30.73,8.13 28.96,8.13 28.19,8.89
  pour Top (no thermals): 16.64,10.67 17.27,10.67 17.27,9.14 17.53,8.89 18.29,8.89 18.54,9.14 18.54,10.67 23.11,10.67 23.11,6.86 21.59,6.86 21.34,6.6 21.34,5.21 21.59,4.95 22.35,4.95 22.35,4.06 20.32,4.06 20.32,6.99 19.18,8.13 17.4,8.13 16.64,8.89
  pour Top (no thermals): 72.52,27.18 83.19,27.18 83.19,23.88 77.85,23.88 77.09,24.64 75.69,24.64 75.69,26.16 73.15,26.16 73.15,24.64 72.52,24.64
VFB1  (via drill 0.25)
  Top 0.203: U1.5 17.27,35.56 17.65,35.18 22.61,35.18 | 22.61,40.09 22.61,40.13 | 22.61,35.18 22.61,40.09 | v22.99,34.42 22.99,35.18 22.61,35.18 | 22.61,40.09 R5.2
  Top 0.254: R5.2 22.57,40.39
  Top 0.406: 22.57,40.39 C1.2 22.61,41.91 22.61,43.05 R1.1
  Bottom 0.203: v22.99,34.42 22.99,34.92 22.61,35.31 21.97,35.31 21.97,35.69 R78.1
VFB2  (via drill 0.25)
  Top 0.203: U2.5 28.83,35.56 29.21,35.18 34.16,35.18 | 34.16,40.09 34.16,40.13 | 34.16,35.18 34.16,40.09 | v34.54,34.42 34.54,35.18 34.16,35.18 | 34.16,40.09 R6.2
  Top 0.254: R6.2 34.12,40.39
  Top 0.406: 34.12,40.39 C2.2 34.16,41.91 34.16,43.05 R2.1
  Bottom 0.203: v34.54,34.42 34.54,34.92 34.16,35.31 33.53,35.31 33.53,35.69 R76.1
VFB3  (via drill 0.25)
  Top 0.203: U3.5 40.39,35.56 40.77,35.18 45.72,35.18 | 45.72,40.09 45.72,40.13 | 45.72,35.18 45.72,40.09 | v46.1,34.42 46.1,35.18 45.72,35.18 | 45.72,40.09 R7.2
  Top 0.254: R7.2 45.68,40.39
  Top 0.406: 45.68,40.39 C3.2 45.72,41.91 45.72,43.05 R3.1
  Bottom 0.203: v46.1,34.42 46.1,34.92 45.72,35.31 45.09,35.31 45.09,35.69 R74.1
VFB4  (via drill 0.25)
  Top 0.203: U9.5 17.91,10.79 17.53,11.18 12.57,11.18 | 12.57,6.26 12.57,6.22 | 12.57,6.26 12.57,11.18 | v12.19,11.94 12.19,11.18 12.57,11.18 | R31.2 12.57,6.26
  Top 0.254: 12.61,5.97 R31.2
  Top 0.406: 12.61,5.97 C28.2 12.57,4.45 12.57,3.3 R37.1
  Bottom 0.203: v12.19,11.94 12.19,11.43 12.57,11.05 13.21,11.05 13.21,10.67 R56.1
VFB5  (via drill 0.25)
  Top 0.203: U10.5 29.46,10.79 29.08,11.18 24.13,11.18 | 24.13,6.26 24.13,6.22 | 24.13,6.26 24.13,11.18 | v23.75,11.94 23.75,11.18 24.13,11.18 | R32.2 24.13,6.26
  Top 0.254: 24.17,5.97 R32.2
  Top 0.406: 24.17,5.97 C29.2 24.13,4.45 24.13,3.3 R38.1
  Bottom 0.203: v23.75,11.94 23.75,11.43 24.13,11.05 24.77,11.05 24.77,10.67 R54.1
VFB6  (via drill 0.25)
  Top 0.203: U11.5 41.02,10.79 40.64,11.18 35.69,11.18 | 35.69,6.26 35.69,6.22 | 35.69,6.26 35.69,11.18 | v35.31,11.94 35.31,11.18 35.69,11.18 | R33.2 35.69,6.26
  Top 0.254: 35.73,5.97 R33.2
  Top 0.406: 35.73,5.97 C30.2 35.69,4.45 35.69,3.3 R39.1
  Bottom 0.203: v35.31,11.94 35.31,11.43 35.69,11.05 36.32,11.05 36.32,10.67 R52.1
VFB7  (via drill 0.25)
  Top 0.203: U12.5 52.58,10.79 52.2,11.18 47.24,11.18 | 47.24,6.26 47.24,6.22 | 47.24,6.26 47.24,11.18 | v46.86,11.94 46.86,11.18 47.24,11.18 | R34.2 47.24,6.26
  Top 0.254: 47.28,5.97 R34.2
  Top 0.406: 47.28,5.97 C31.2 47.24,4.45 47.24,3.3 R40.1
  Bottom 0.203: v46.86,11.94 46.86,11.43 47.24,11.05 47.88,11.05 47.88,10.67 R50.1
VFB12  (via drill 0.25)
  Top 0.203: U4.5 51.94,35.56 52.32,35.18 57.28,35.18 | 57.28,40.09 57.28,40.13 | 57.28,35.18 57.28,40.09 | v57.66,34.42 57.66,35.18 57.28,35.18 | 57.28,40.09 R8.2
  Top 0.254: R8.2 57.24,40.39
  Top 0.406: 57.24,40.39 C4.2 57.28,41.91 57.28,43.05 R4.1
  Bottom 0.203: v57.66,34.42 57.66,34.92 57.28,35.31 56.64,35.31 56.64,35.69 R72.1
VOUT_CH0
  Top 0.254: R1.2 20.87,43.05 C1.1 17.4,41.91 TP3.TP
  pour Top (no thermals): 22.1,35.69 19.05,35.69 19.05,37.72 18.03,38.73 16.26,38.73 15.37,39.62 15.37,42.42 17.02,44.07 21.34,44.07 21.34,41.4 19.81,41.4 18.92,40.51 18.92,39.88 19.56,39.24 22.1,39.24
  pour Bottom (no thermals): 23.37,44.07 23.37,41.78 20.19,41.78 18.92,40.51 18.92,37.21 18.41,36.7 18.41,35.05 16.89,35.05 16,35.94 12.45,35.94 12.19,36.2 12.19,37.85 14.73,37.85 15.11,38.23 15.11,42.16 17.02,44.07
VOUT_CH1
  Top 0.254: R2.2 32.42,43.05 C2.1 28.96,41.91 TP4.TP
  pour Top (no thermals): 33.66,35.69 30.61,35.69 30.61,37.72 29.59,38.73 27.81,38.73 26.92,39.62 26.92,42.42 28.57,44.07 32.89,44.07 32.89,41.4 31.37,41.4 30.48,40.51 30.48,39.88 31.11,39.24 33.66,39.24
  pour Bottom (no thermals): 34.92,44.07 34.92,41.78 31.75,41.78 30.48,40.51 30.48,37.21 29.97,36.7 29.97,35.05 28.45,35.05 27.56,35.94 24,35.94 23.75,36.2 23.75,37.85 26.29,37.85 26.67,38.23 26.67,42.16 28.57,44.07
VOUT_CH2
  Top 0.254: R3.2 43.98,43.05 C3.1 40.51,41.91 TP5.TP
  pour Top (no thermals): 45.21,35.69 42.16,35.69 42.16,37.72 41.15,38.73 39.37,38.73 38.48,39.62 38.48,42.42 40.13,44.07 44.45,44.07 44.45,41.4 42.93,41.4 42.04,40.51 42.04,39.88 42.67,39.24 45.21,39.24
  pour Bottom (no thermals): 46.48,44.07 46.48,41.78 43.31,41.78 42.04,40.51 42.04,37.21 41.53,36.7 41.53,35.05 40.01,35.05 39.12,35.94 35.56,35.94 35.31,36.2 35.31,37.85 37.85,37.85 38.23,38.23 38.23,42.16 40.13,44.07
VOUT_CH3
  Top 0.254: R4.2 55.54,43.05 C4.1 52.07,41.91 TP6.TP
  pour Top (no thermals): 56.77,35.69 53.72,35.69 53.72,37.72 52.7,38.73 50.93,38.73 50.04,39.62 50.04,42.42 51.69,44.07 56.01,44.07 56.01,41.4 54.48,41.4 53.59,40.51 53.59,39.88 54.23,39.24 56.77,39.24
  pour Bottom (no thermals): 58.04,44.07 58.04,41.78 54.86,41.78 53.59,40.51 53.59,37.21 53.09,36.7 53.09,35.05 51.56,35.05 50.67,35.94 47.12,35.94 46.86,36.2 46.86,37.85 49.4,37.85 49.78,38.23 49.78,42.16 51.69,44.07
VOUT_CH4
  Top 0.254: R37.2 14.31,3.3 C28.1 17.78,4.45 TP17.TP
  pour Top (no thermals): 13.08,10.67 16.13,10.67 16.13,8.64 17.14,7.62 18.92,7.62 19.81,6.73 19.81,3.94 18.16,2.29 13.84,2.29 13.84,4.95 15.37,4.95 16.26,5.84 16.26,6.48 15.62,7.11 13.08,7.11
  pour Bottom (no thermals): 11.81,2.29 11.81,4.57 14.99,4.57 16.26,5.84 16.26,9.14 16.76,9.65 16.76,11.3 18.29,11.3 19.18,10.41 22.73,10.41 22.99,10.16 22.99,8.51 20.45,8.51 20.07,8.13 20.07,4.19 18.16,2.29
VOUT_CH5
  Top 0.254: R38.2 25.87,3.3 C29.1 29.34,4.45 TP18.TP
  pour Top (no thermals): 24.64,10.67 27.69,10.67 27.69,8.64 28.7,7.62 30.48,7.62 31.37,6.73 31.37,3.94 29.72,2.29 25.4,2.29 25.4,4.95 26.92,4.95 27.81,5.84 27.81,6.48 27.18,7.11 24.64,7.11
  pour Bottom (no thermals): 23.62,2.29 23.62,4.57 26.54,4.57 27.81,5.84 27.81,9.14 28.32,9.65 28.32,11.3 29.84,11.3 30.73,10.41 34.29,10.41 34.54,10.16 34.54,8.51 32,8.51 31.62,8.13 31.62,4.19 29.72,2.29
VOUT_CH6
  Top 0.254: R39.2 37.43,3.3 C30.1 40.89,4.45 TP19.TP
  Bottom 0.406: 41.53,10.67 40.42,10.67 R51.1
  pour Top (no thermals): 36.2,10.67 39.24,10.67 39.24,8.64 40.26,7.62 42.04,7.62 42.93,6.73 42.93,3.94 41.27,2.29 36.96,2.29 36.96,4.95 38.48,4.95 39.37,5.84 39.37,6.48 38.73,7.11 36.2,7.11
  pour Bottom (no thermals): 35.18,2.29 35.18,4.57 38.1,4.57 39.37,5.84 39.37,9.14 39.88,9.65 39.88,11.3 41.4,11.3 42.29,10.41 45.85,10.41 46.1,10.16 46.1,8.51 43.56,8.51 43.18,8.13 43.18,4.19 41.27,2.29
VOUT_CH7
  Top 0.254: R40.2 48.98,3.3 C31.1 52.45,4.45 TP20.TP
  pour Top (no thermals): 47.75,10.67 50.8,10.67 50.8,8.64 51.82,7.62 53.59,7.62 54.48,6.73 54.48,3.94 52.83,2.29 48.51,2.29 48.51,4.95 50.04,4.95 50.93,5.84 50.93,6.48 50.29,7.11 47.75,7.11
  pour Bottom (no thermals): 46.74,2.29 46.74,4.57 49.66,4.57 50.93,5.84 50.93,9.14 51.44,9.65 51.44,11.3 52.96,11.3 53.85,10.41 57.4,10.41 57.66,10.16 57.66,8.51 55.12,8.51 54.74,8.13 54.74,4.19 52.83,2.29
VREF
  Bottom 0.406: U15.6 67.29,22.54 R63.2 67.44,22.35 67.44,24 C43.2
VSNSP_CH0  (via drill 0.25)
  Top 0.203: U6.36 55.41,21.75 v55.75,22.1
  Route15 0.203: v55.75,22.1 55.12,22.1 55.12,22.48 54.48,23.11 54.48,23.75 53.34,24.89 48.13,24.89 47.37,25.65 42.55,25.65 41.15,27.05 33.27,27.05 32.38,27.94 32.38,30.23 31.5,31.11 29.34,31.11 28.45,30.23 27.69,30.23 26.8,31.11 21.72,31.11 20.57,32.26 VSNSN24.1
  Bottom 0.203: 17.91,33.91 R79.2 | 19.56,33.91 C53.2
  Bottom 0.406: VSNSN24.1 19.56,33.91 17.91,33.91
VSNSP_CH1  (via drill 0.25)
  Top 0.203: U6.42 55.74,24.75 55.88,24.89 v55.88,25.02
  Route15 0.203: v55.88,25.02 55.24,25.02 54.23,26.04 48.9,26.04 47.12,27.81 43.81,27.81 43.43,28.19 34.16,28.19 33.66,28.7 33.66,31.5 34.16,32 34.16,32.64 33.66,33.15 32,33.15 VSNSN22.1
  Bottom 0.203: 29.46,33.91 R77.2 | 31.11,33.91 C52.2
  Bottom 0.406: VSNSN22.1 31.11,33.91 29.46,33.91
VSNSP_CH2  (via drill 0.25)
  Top 0.203: U6.46 55.45,26.75 55.63,26.92 56.52,26.92 56.77,26.67 v56.77,26.29
  Route15 0.203: v56.77,26.29 56.77,26.67 56.52,26.92 49.28,26.92 47.88,28.32 47.88,29.84 45.72,32 45.72,32.64 45.34,33.02 44.45,33.02 43.69,32.26 VSNSN20.1
  Bottom 0.203: 41.02,33.91 R75.2 | 42.67,33.91 C51.2
  Bottom 0.406: VSNSN20.1 42.67,33.91 41.02,33.91
VSNSP_CH3  (via drill 0.25)
  Top 0.203: U6.48 54.8,27.75 54.86,27.81 v54.86,28.7
  Bottom 0.203: 52.58,33.91 R73.2 | 54.23,33.91 C50.2 | v54.86,28.7 55.12,28.7 55.12,31.88 54.74,32.26 VSNSN18.1
  Bottom 0.406: VSNSN18.1 54.23,33.91 52.58,33.91
VSNSP_CH4  (via drill 0.25)
  Top 0.203: U6.52 52.54,29.05 53.21,29.72 55.75,29.72 56.52,28.96 56.52,28.45 55.75,27.69 v55.75,27.56
  Route15 0.203: v55.75,27.56 55.75,27.69 56.26,28.19 57.91,28.19 58.17,27.94 58.17,22.1 56.39,20.32 47.12,20.32 45.21,22.23 44.45,22.23 44.07,21.84 44.07,18.8 43.56,18.29 40.39,18.29 39.24,19.43 26.8,19.43 26.67,19.3 25.4,19.3 25.27,19.43 v25.27,19.94
  Bottom 0.203: 17.27,12.45 R55.2 17.53,12.66 17.53,14.99 17.78,15.24 24.77,15.24 25.27,15.75 v25.27,19.94 | C40.2 15.62,12.45
  Bottom 0.406: VSNSN15.1 15.62,12.45 17.27,12.45
VSNSP_CH5  (via drill 0.25)
  Top 0.203: U6.62 47.54,29.17 47.37,29.34 46.1,29.34 45.72,28.96 44.96,28.96 v44.45,28.45
  Bottom 0.203: 28.83,12.45 R53.2 | C39.2 27.18,12.45 | v44.45,28.45 44.2,28.19 42.93,28.19 42.55,27.81 42.55,26.8 43.05,26.29 43.05,15.88 42.67,15.49 39.5,15.49 38.86,14.86 29.84,14.86 28.96,13.97 27.3,13.97 VSNSN13.1
  Bottom 0.406: VSNSN13.1 27.18,12.45 28.83,12.45
VSNSP_CH6  (via drill 0.25)
  Top 0.203: U6.64 45.39,28.5 44.7,27.81 43.56,27.81 43.43,27.69 43.43,27.43 v43.18,27.43
  Bottom 0.203: 40.39,12.45 R51.2 | C38.2 38.73,12.45 | v43.18,27.43 43.43,27.43 43.43,15.24 43.18,14.99 39.62,14.99 VSNSN11.1
  Bottom 0.406: VSNSN11.1 38.73,12.45 40.39,12.45
VSNSP_CH7  (via drill 0.25)
  Top 0.203: U6.2 44.52,27.25 v44.45,27.18
  Bottom 0.203: 51.94,12.45 R49.2 | C37.2 50.29,12.45 | v44.45,27.18 44.2,27.18 44.2,15.62 44.45,15.37 48.26,15.37 49.53,14.1 VSNSN9.1
  Bottom 0.406: VSNSN9.1 50.29,12.45 51.94,12.45

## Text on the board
tPlace: CH0 1.2V | CH1 1.5V | CH2 1.8V | CH3 2.0V | GND | INSTALL CONNECTORS | ON TOP SIDE | F | E | M | A | L | E | GND | 6-14V | 0.3A | 0.3A | 0.3A | 0.3A | FAULT | - | + | SHARE_CLK | CONTROL | ALERT | RESET | LTC2977CUP | DEMO CIRCUIT 2028A | FAULT | SCL | GND | GND | ALERT | 8-CHANNEL POWER | +5V | SHORT | SYSTEM MANAGER | RUN | OFF | SDA | CONTROL | 0.3A | 0.3A | 0.3A | 0.3A | M | A | L | E | GND | CH4 2.5V | CH5 2.7V | CH6 3.0V | CH7 3.3V
bPlace: CH0 1.2V | CH1 1.5V | CH2 1.8V | CH3 2.0V | REV 1 | RUN | VS | DAC | RUN | VS | DAC | RUN | VS | DAC | RUN | VS | DAC | LTC CONFIDENTIAL | FOR CUSTOMER USE | ONLY | VS | DAC | VS | RUN | DAC | VS | RUN | DAC | VS | RUN | DAC | RUN | HI | LO | A2 | A1 | A0 | 1 | CH4 2.5V | CH5 2.7V | CH6 3.0V | CH7 3.3V
tStop: LTC2977CUP | 8-CHANNEL | POWER MANAGER | (408) 432-1900 | www.linear.com
bStop: POWER MANAGER | 8-CHANNEL | LTC2977CUP | (408) 432-1900 | www.linear.com
d_FabDrawing: 1.825" | DRILL TABLE | 0.00" | 0.00" | 3.365" | SHOWN FROM TOP SIDE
